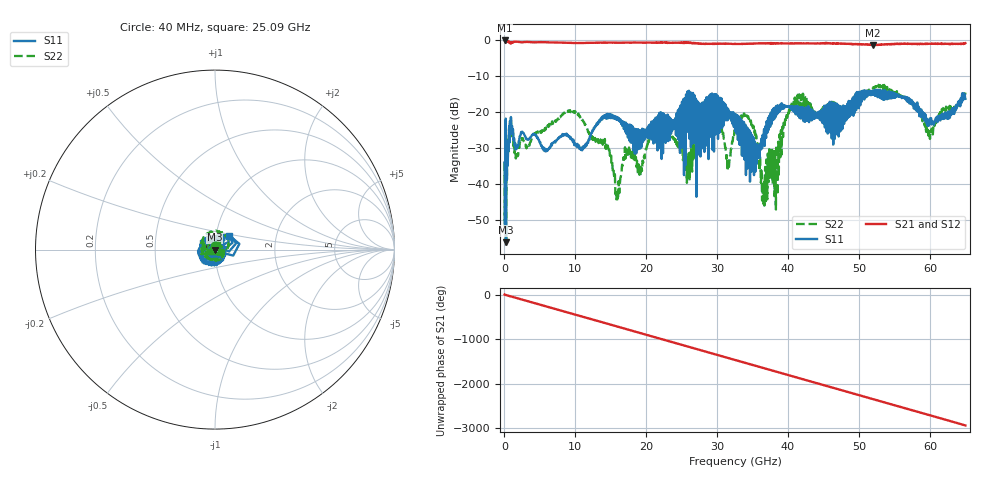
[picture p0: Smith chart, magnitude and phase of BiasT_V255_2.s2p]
! Created Tue Jul 15 19:49:50 2008
# hz S ma R 50
! 2 Port Network Data from blockName block
! freq  magS11  angS11  magS21  angS21  magS12  angS12  magS22  angS22
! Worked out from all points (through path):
!   1601 points, 40 MHz to 65 GHz, reference 50 ohm
!   highest |S21| = -0.03 dB at 80.6 MHz (marker M1); lowest = -1.3 dB at 52.01 GHz (marker M2)
!   group delay of S21, straight-line fit = 125 ps
!   lowest |S11| = -56.3 dB at 243 MHz (marker M3), VSWR 1.00, Z = 49.8 - j0.0243 ohm
!   |S11| at or under -10 dB: start of sweep to end of sweep
!   |S22| runs from -57.4 to -12.4 dB; largest |S21 - S12| = 0.042
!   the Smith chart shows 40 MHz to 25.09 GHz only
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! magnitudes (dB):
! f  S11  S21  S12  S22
! 40 MHz  -34.0  -0.1  -0.1  -34.0
! 80.6 MHz  -51.1  0.0  0.0  -51.9
! 243 MHz  -56.3  -0.1  -0.1  -57.4
! 973.8 MHz  -24.0  -0.7  -0.7  -24.5
! 10.88 GHz  -30.0  -0.7  -0.7  -21.6
! 14.49 GHz  -20.7  -0.6  -0.6  -30.2
! 15.96 GHz  -22.2  -0.7  -0.6  -43.4
! 17.09 GHz  -24.0  -0.6  -0.6  -32.9
! 19.12 GHz  -27.4  -0.6  -0.6  -35.2
! 21.72 GHz  -21.4  -0.6  -0.6  -24.2
! 25.82 GHz  -14.3  -0.7  -0.6  -32.0
! 28.87 GHz  -15.4  -1.0  -1.0  -22.3
! 31.55 GHz  -19.1  -0.9  -1.0  -33.8
! 32.52 GHz  -23.6  -1.0  -1.0  -25.1
! 34.63 GHz  -39.4  -0.9  -0.9  -22.5
! 36.54 GHz  -28.2  -0.8  -0.8  -45.6
! 40.64 GHz  -19.6  -0.8  -0.8  -19.1
! 43.36 GHz  -21.8  -0.8  -0.9  -18.2
! 52.01 GHz  -14.5  -1.3  -1.3  -13.1
! 54.2 GHz  -15.1  -1.0  -1.1  -13.7
! 60.09 GHz  -22.5  -1.0  -1.0  -26.2
! 65 GHz  -16.3  -0.8  -1.2  -14.5
